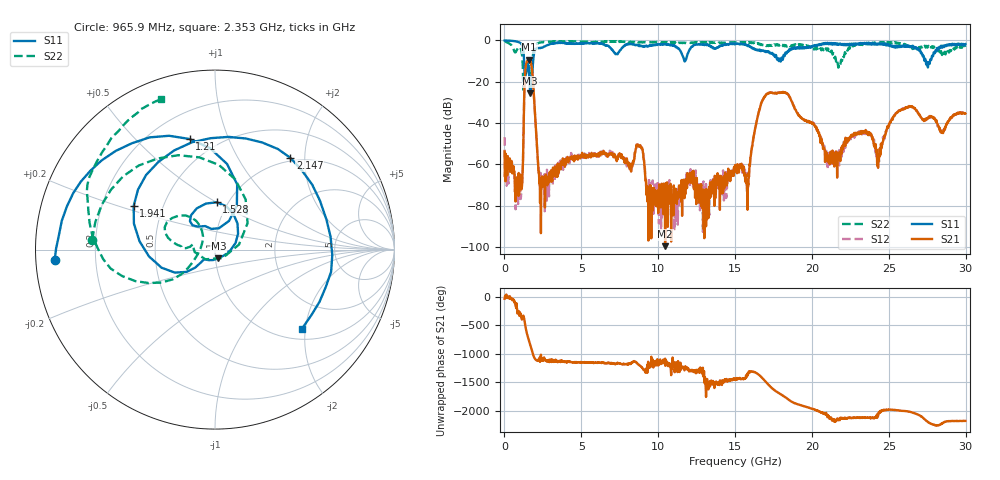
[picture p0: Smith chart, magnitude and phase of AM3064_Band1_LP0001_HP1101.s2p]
# Hz S DB R 50.0
!freq dBS11 angS11 dBS21 angS21 dBS12 angS12 dBS22 angS22
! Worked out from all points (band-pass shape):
!   1600 points, 10 MHz to 29.98 GHz, reference 50 ohm
!   highest |S21| = -9.41 dB at 1.603 GHz (marker M1); lowest = -99.7 dB at 10.45 GHz (marker M2)
!   |S21| within 3 dB of the highest: 1.387 GHz to 1.761 GHz (373.6 MHz wide, 23.7 % of centre)
!   lowest |S11| = -25.6 dB at 1.678 GHz (marker M3), VSWR 1.11, Z = 51.6 - j5.07 ohm
!   |S11| at or under -10 dB: 1.277 GHz to 1.866 GHz (589.8 MHz wide, 37.5 % of centre); 11.70386 GHz to 11.75181 GHz (47.95 MHz wide, 0.409 % of centre); 27.4 GHz to 27.68 GHz (282.3 MHz wide, 1.03 % of centre)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
!   |S22| runs from -23.9 to -0.2 dB; largest |S21 - S12| = 0.0059
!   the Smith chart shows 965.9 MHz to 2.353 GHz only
!   S11 on the Smith chart (normalised r, x): 965.9 MHz: 0.06, -0.03; 1.21 GHz: 0.36, +0.73; 1.528 GHz: 0.88, +0.50; 1.941 GHz: 0.34, +0.22; 2.147 GHz: 0.94, +1.71; 2.353 GHz: 1.23, -1.91
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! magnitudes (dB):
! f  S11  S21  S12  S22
! 10 MHz  0.0  -53.8  -46.8  -0.2
! 965.9 MHz  -1.0  -69.0  -67.2  -3.3
! 1.21 GHz  -4.0  -57.5  -56.2  -17.3
! 1.528 GHz  -11.6  -9.6  -9.5  -10.2
! 1.603 GHz  -16.1  -9.4  -9.4  -13.1
! 1.678 GHz  -25.6  -9.9  -9.9  -20.1
! 1.941 GHz  -5.8  -30.0  -29.9  -3.7
! 2.147 GHz  -3.6  -54.8  -55.5  -1.5
! 2.353 GHz  -3.7  -68.6  -64.2  -1.0
! 5.015 GHz  -1.4  -56.4  -56.3  -0.6
! 8.801 GHz  -2.6  -51.3  -51.0  -0.9
! 9.363 GHz  -2.8  -96.9  -77.8  -0.9
! 10 GHz  -2.0  -83.6  -74.9  -0.9
! 10.45 GHz  -1.8  -99.7  -71.0  -1.0
! 15 GHz  -1.7  -60.4  -61.4  -1.3
! 15.81 GHz  -2.7  -82.0  -70.6  -1.2
! 17.14 GHz  -5.7  -25.6  -25.6  -2.7
! 19.99 GHz  -3.3  -40.1  -40.2  -3.3
! 21.12 GHz  -1.3  -59.6  -60.2  -4.9
! 24.32 GHz  -1.9  -56.6  -58.0  -1.0
! 25 GHz  -2.0  -40.8  -41.0  -1.2
! 29.98 GHz  -1.8  -35.4  -35.6  -3.2
